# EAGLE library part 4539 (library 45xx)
Dual 4-channel DATA SELECTOR/MULTIPLEXER
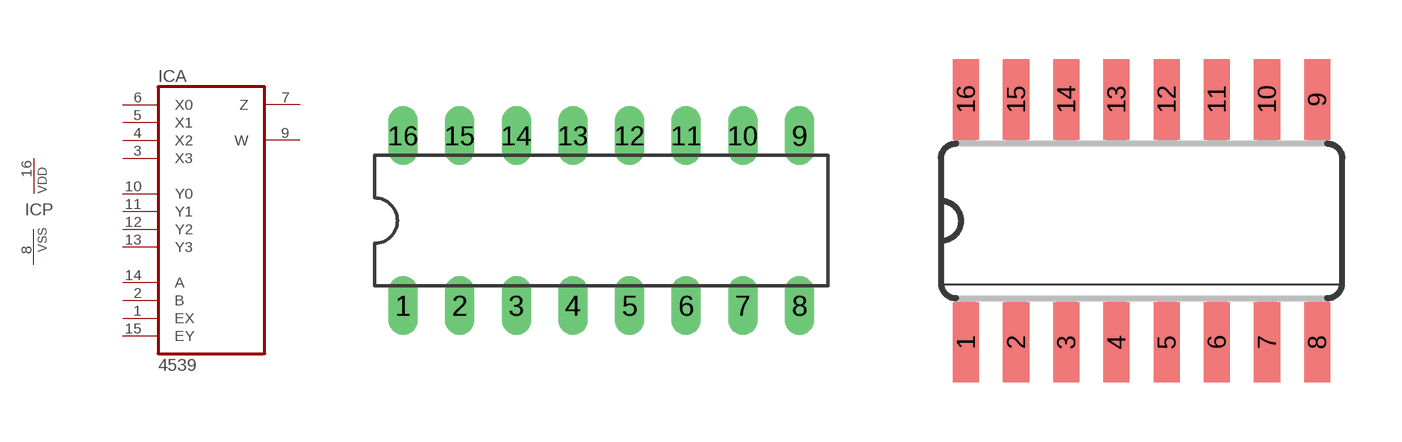
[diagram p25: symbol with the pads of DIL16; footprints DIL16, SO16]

Designator prefix IC; gates A=4539 P=PWRN

## 4539N  [DIL16]
1  A:EX  in
2  A:B  in
3  A:X3  in
4  A:X2  in
5  A:X1  in
6  A:X0  in
7  A:Z  hiz
8  P:VSS  pwr
9  A:W  hiz
10  A:Y0  in
11  A:Y1  in
12  A:Y2  in
13  A:Y3  in
14  A:A  in
15  A:EY  in
16  P:VDD  pwr

## 4539D  [SO16]
Pads as for DIL16

## Footprint DIL16 (pad centres in mm)
Dual In Line Package
drill 0.813 long: 1 -8.89,-3.81; 2 -6.35,-3.81; 3 -3.81,-3.81; 4 -1.27,-3.81; 5 1.27,-3.81; 6 3.81,-3.81; 7 6.35,-3.81; 8 8.89,-3.81; 9 8.89,3.81; 10 6.35,3.81; 11 3.81,3.81; 12 1.27,3.81; 13 -1.27,3.81; 14 -3.81,3.81; 15 -6.35,3.81; 16 -8.89,3.81

## Footprint SO16 (pad centres in mm)
Small Outline package 150 mil
smd 0.66 x 2.032: 1 -4.445,-3.073; 2 -3.175,-3.073; 3 -1.905,-3.073; 4 -0.635,-3.073; 5 0.635,-3.073; 6 1.905,-3.073; 7 3.175,-3.073; 8 4.445,-3.073; 9 4.445,3.073; 10 3.175,3.073; 11 1.905,3.073; 12 0.635,3.073; 13 -0.635,3.073; 14 -1.905,3.073; 15 -3.175,3.073; 16 -4.445,3.073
